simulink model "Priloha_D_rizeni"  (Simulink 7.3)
settings: Solver=ode45  StartTime=0.0  StopTime=0.7  FixedStep=0.6e-3  MaxStep=0.08e-3  RelTol=0.8e-3
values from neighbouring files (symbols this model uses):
  ILi = [0 Imax]    [Priloha_B_motor1_parametry.m]    (also in Priloha_C_motor2_parametry.m)
  Im = Psim / Ldi(1)    [Priloha_B_motor1_parametry.m]    (also in Priloha_C_motor2_parametry.m)
  Imax = 8    [Priloha_B_motor1_parametry.m]    (also in Priloha_C_motor2_parametry.m)
  J = 7e-3    (= 0.007)    [Priloha_B_motor1_parametry.m]    (also in Priloha_C_motor2_parametry.m)
  Kiid = 1 / (KM * 2 * tausigmaid / Rs)    (= 1975)    [Priloha_B_motor1_parametry.m]    (also in Priloha_C_motor2_parametry.m)
  Kiiq = 1 / (KM * 2 * tausigmaiq / Rs)    (= 1975)    [Priloha_B_motor1_parametry.m]    (also in Priloha_C_motor2_parametry.m)
  Kiwq = 1 / (Psim * p * 8 * (2 * tausigmaiq)^2 / J)    (= 306.115309264)    [Priloha_B_motor1_parametry.m]    (also in Priloha_C_motor2_parametry.m = 402.854511971)
  KM = 1    [Priloha_B_motor1_parametry.m]    (also in Priloha_C_motor2_parametry.m)
  Kpid = Ldi(1) / (KM * 2 * tausigmaid)    [Priloha_B_motor1_parametry.m]    (also in Priloha_C_motor2_parametry.m)
  Kpiq = Lqi(1) / (KM * 2 * tausigmaiq)    [Priloha_B_motor1_parametry.m]    (also in Priloha_C_motor2_parametry.m)
  Kpwq = 4 / (Psim * p * 8 * (2 * tausigmaiq) / J)    (= 2.44892247411)    [Priloha_B_motor1_parametry.m]    (also in Priloha_C_motor2_parametry.m = 3.22283609576)
  Ld = 22.5e-3    (= 0.0225)    [Priloha_B_motor1_parametry.m]    (also in Priloha_C_motor2_parametry.m)
  Ldi = [Ldi Ldi]    [Priloha_B_motor1_parametry.m]    (also in Priloha_C_motor2_parametry.m)
  Lq = 54e-3    (= 0.054)    [Priloha_B_motor1_parametry.m]    (also in Priloha_C_motor2_parametry.m)
  Lqi = [Lqi Lqi]    [Priloha_B_motor1_parametry.m]    (also in Priloha_C_motor2_parametry.m)
  p = 3    [Priloha_B_motor1_parametry.m]    (also in Priloha_C_motor2_parametry.m)
  Psim = 238.2e-3    (= 0.2382)    [Priloha_B_motor1_parametry.m]    (also in Priloha_C_motor2_parametry.m = 0.181)
  Rs = 3.95    [Priloha_B_motor1_parametry.m]    (also in Priloha_C_motor2_parametry.m)
  tausigmaid = 1 / fM    (= 0.001)    [Priloha_B_motor1_parametry.m]    (also in Priloha_C_motor2_parametry.m)
  tausigmaiq = 1 / fM    (= 0.001)    [Priloha_B_motor1_parametry.m]    (also in Priloha_C_motor2_parametry.m)
  Umax = 115    [Priloha_B_motor1_parametry.m]    (also in Priloha_C_motor2_parametry.m)
undefined symbols (not defined in the file or in its folder): Floor, magnitude
libraries: simulink x21
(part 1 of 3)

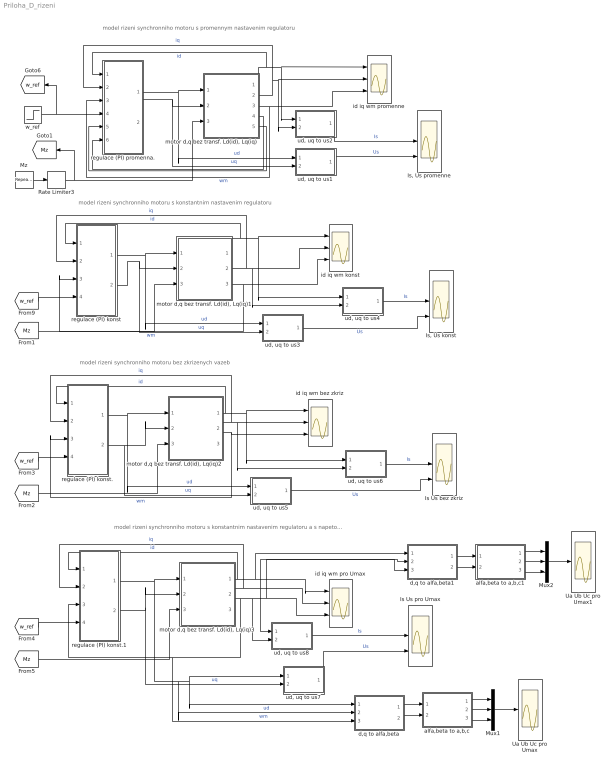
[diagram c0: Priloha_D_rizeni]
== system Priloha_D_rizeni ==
  note: model rizeni synchronniho motoru s promennym nastavenim regulatoru
  note: model rizeni synchronniho motoru s konstantnim nastavenim regulatoru
  note: model rizeni synchronniho motoru bez zkrizenych vazeb
  note: model rizeni synchronniho motoru s konstantnim nastavenim regulatoru a s napetovym omezenim
  Is Us bez zkriz : Scope  NumInputPorts=3
  Is Us pro Umax : Scope  NumInputPorts=3
  "Is, Us konst" : Scope  NumInputPorts=3
  "Is, Us promenne" : Scope  NumInputPorts=3
  Mux1 : Mux  Inputs=3
  Mux2 : Mux  Inputs=3
  Mz : simulink/Sources/Repeating Sequence Stair  SystemSampleTime=-1  OutValues=[0 0 0 4.0 4.0 4.0 0 0]  tsamp=0.1  OutMin=[]  OutMax=[]  OutDataTypeStr=double  OutputDataTypeScalingMode=Specify via dialog  OutDataType=double  ConRadixGroup=Best Precision: Vector-wise  OutScaling=2^-12
  Rate Limiter3 : RateLimiter  RisingSlewLimit=1000  FallingSlewLimit=-200000
  Ua Ub Uc pro Umax : Scope  NumInputPorts=3
  Ua Ub Uc pro Umax1 : Scope  NumInputPorts=3
  alfa,beta to a,b,c : Subsystem
  alfa,beta to a,b,c1 : Subsystem
  d,q to alfa,beta : Subsystem
  d,q to alfa,beta1 : Subsystem
  id iq wm bez zkriz : Scope  NumInputPorts=3
  id iq wm konst : Scope  NumInputPorts=3
  id iq wm pro Umax : Scope  NumInputPorts=3
  id iq wm promenne : Scope  NumInputPorts=3
  "motor d,q bez transf. Ld(id), Lq(iq)" : Subsystem
  "motor d,q bez transf. Ld(id), Lq(iq)1" : Subsystem
  "motor d,q bez transf. Ld(id), Lq(iq)2" : Subsystem
  "motor d,q bez transf. Ld(id), Lq(iq)3" : Subsystem
  regulace (PI) konst : Subsystem
  regulace (PI) konst. : Subsystem
  regulace (PI) konst.1 : Subsystem
  regulace (PI) promenna. : Subsystem
  "ud, uq to us1" : Subsystem
  "ud, uq to us2" : Subsystem
  "ud, uq to us3" : Subsystem
  "ud, uq to us4" : Subsystem
  "ud, uq to us5" : Subsystem
  "ud, uq to us6" : Subsystem
  "ud, uq to us7" : Subsystem
  "ud, uq to us8" : Subsystem
  w_ref : Step  Time=0.01  After=130  SampleTime=0
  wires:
  "ud, uq to us2"/1(is) -> "Is, Us promenne"/2  "Is"
  "motor d,q bez transf. Ld(id), Lq(iq)"/1(id) -> regulace (PI) promenna./1(id1), id iq wm promenne/1, "ud, uq to us2"/1(id)  "id"
  "motor d,q bez transf. Ld(id), Lq(iq)"/2(iq) -> regulace (PI) promenna./2(iq1), id iq wm promenne/2, "ud, uq to us2"/2(iq)  "iq"
  "motor d,q bez transf. Ld(id), Lq(iq)"/3(wm) -> id iq wm promenne/3, regulace (PI) promenna./3(wm2)  "wm"
  regulace (PI) promenna./1(ud) -> "motor d,q bez transf. Ld(id), Lq(iq)"/1(ud), "ud, uq to us1"/1(ud)  "ud"
  regulace (PI) promenna./2(uq) -> "motor d,q bez transf. Ld(id), Lq(iq)"/2(uq), "ud, uq to us1"/2(uq)  "uq"
  "ud, uq to us1"/1(us) -> "Is, Us promenne"/3  "Us"
  "motor d,q bez transf. Ld(id), Lq(iq)"/4(Ld) -> regulace (PI) promenna./6(Ld)
  "motor d,q bez transf. Ld(id), Lq(iq)"/5(Lq) -> regulace (PI) promenna./5(Lq)
  w_ref/1 -> regulace (PI) promenna./4(w_ref), [w_ref]
  Mz/1 -> Rate Limiter3/1
  Rate Limiter3/1 -> "motor d,q bez transf. Ld(id), Lq(iq)"/3(Mm), [Mz]
  "ud, uq to us4"/1(is) -> "Is, Us konst"/2  "Is"
  "motor d,q bez transf. Ld(id), Lq(iq)1"/1(id) -> regulace (PI) konst/1(id1), id iq wm konst/1, "ud, uq to us4"/1(id)  "id"
  "motor d,q bez transf. Ld(id), Lq(iq)1"/2(iq) -> id iq wm konst/2, "ud, uq to us4"/2(iq), regulace (PI) konst/2(iq1)  "iq"
  "motor d,q bez transf. Ld(id), Lq(iq)1"/3(wm) -> regulace (PI) konst/3(wm2), id iq wm konst/3  "wm"
  regulace (PI) konst/1(ud) -> "motor d,q bez transf. Ld(id), Lq(iq)1"/1(ud), "ud, uq to us3"/1(ud)  "ud"
  regulace (PI) konst/2(uq) -> "motor d,q bez transf. Ld(id), Lq(iq)1"/2(uq), "ud, uq to us3"/2(uq)  "uq"
  "ud, uq to us3"/1(us) -> "Is, Us konst"/3  "Us"
  [w_ref] -> regulace (PI) konst/4(w_ref)
  [Mz] -> "motor d,q bez transf. Ld(id), Lq(iq)1"/3(Mm)
  "ud, uq to us6"/1(is) -> Is Us bez zkriz/2  "Is"
  "motor d,q bez transf. Ld(id), Lq(iq)2"/1(id) -> id iq wm bez zkriz/1, "ud, uq to us6"/1(id), regulace (PI) konst./1(id)  "id"
  "motor d,q bez transf. Ld(id), Lq(iq)2"/2(iq) -> id iq wm bez zkriz/2, "ud, uq to us6"/2(iq), regulace (PI) konst./2(iq)  "iq"
  "motor d,q bez transf. Ld(id), Lq(iq)2"/3(wm) -> regulace (PI) konst./3(wm), id iq wm bez zkriz/3  "wm"
  regulace (PI) konst./1(ud) -> "motor d,q bez transf. Ld(id), Lq(iq)2"/1(ud), "ud, uq to us5"/1(ud)  "ud"
  regulace (PI) konst./2(uq) -> "motor d,q bez transf. Ld(id), Lq(iq)2"/2(uq), "ud, uq to us5"/2(uq)  "uq"
  "ud, uq to us5"/1(us) -> Is Us bez zkriz/3  "Us"
  [Mz] -> "motor d,q bez transf. Ld(id), Lq(iq)2"/3(Mm)
  [w_ref] -> regulace (PI) konst./4(w_ref)
  "ud, uq to us8"/1(is) -> Is Us pro Umax/2  "Is"
  "motor d,q bez transf. Ld(id), Lq(iq)3"/1(id) -> regulace (PI) konst.1/1(id1), id iq wm pro Umax/1, d,q to alfa,beta1/1(d)  "id"
  "motor d,q bez transf. Ld(id), Lq(iq)3"/2(iq) -> id iq wm pro Umax/2, "ud, uq to us8"/1(id), d,q to alfa,beta1/2(q), regulace (PI) konst.1/2(iq1)  "iq"
  "motor d,q bez transf. Ld(id), Lq(iq)3"/3(wm) -> "ud, uq to us8"/2(iq), id iq wm pro Umax/3, d,q to alfa,beta1/3(wm), regulace (PI) konst.1/3(wm2), d,q to alfa,beta/3(wm)  "wm"
  "ud, uq to us7"/1(us) -> Is Us pro Umax/3  "Us"
  d,q to alfa,beta/1(alfa) -> alfa,beta to a,b,c/1(alfa)
  d,q to alfa,beta/2(beta) -> alfa,beta to a,b,c/2(beta)
  alfa,beta to a,b,c/1(a) -> Mux1/1
  alfa,beta to a,b,c/2(b) -> Mux1/2
  alfa,beta to a,b,c/3(c) -> Mux1/3
  Mux1/1 -> Ua Ub Uc pro Umax/2
  regulace (PI) konst.1/1(ud) -> "motor d,q bez transf. Ld(id), Lq(iq)3"/1(ud), "ud, uq to us7"/1(ud), d,q to alfa,beta/1(d), d,q to alfa,beta/2(q)  "ud"
  regulace (PI) konst.1/2(uq) -> "motor d,q bez transf. Ld(id), Lq(iq)3"/2(uq), "ud, uq to us7"/2(uq)  "uq"
  [w_ref] -> regulace (PI) konst.1/4(w_ref)
  [Mz] -> "motor d,q bez transf. Ld(id), Lq(iq)3"/3(Mm)
  d,q to alfa,beta1/1(alfa) -> alfa,beta to a,b,c1/1(alfa)
  d,q to alfa,beta1/2(beta) -> alfa,beta to a,b,c1/2(beta)
  alfa,beta to a,b,c1/1(a) -> Mux2/1
  alfa,beta to a,b,c1/2(b) -> Mux2/2
  alfa,beta to a,b,c1/3(c) -> Mux2/3
  Mux2/1 -> Ua Ub Uc pro Umax1/2

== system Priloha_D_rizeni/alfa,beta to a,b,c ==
  note: transformace alfa, beta do a, b, c
  alfa : Inport  OutDataType=fixdt(1, 16)  OutScaling=2^0
  beta : Inport  Port=2  OutDataType=fixdt(1, 16)  OutScaling=2^0
  Add1 : Sum  Inputs=--  OutDataType=fixdt(1, 16)  OutScaling=2^-10
  Add5 : Sum  Inputs=-+  OutDataType=fixdt(1, 16)  OutScaling=2^-10
  Gain1 : Gain  Gain=1/2  ParameterDataType=fixdt(1, 16)  ParameterScaling=2^0  OutDataType=fixdt(1, 16)  OutScaling=2^0
  Gain2 : Gain  Gain=sqrt(3)/2  ParameterDataType=fixdt(1, 16)  ParameterScaling=2^0  OutDataType=fixdt(1, 16)  OutScaling=2^0
  a : Outport  OutDataType=fixdt(1, 16)  OutScaling=2^0
  b : Outport  Port=2  OutDataType=fixdt(1, 16)  OutScaling=2^0
  c : Outport  Port=3  OutDataType=fixdt(1, 16)  OutScaling=2^0
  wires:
  alfa/1 -> a/1, Gain1/1
  Gain1/1 -> Add5/1, Add1/1
  Add5/1 -> b/1
  beta/1 -> Gain2/1
  Add1/1 -> c/1
  Gain2/1 -> Add5/2, Add1/2

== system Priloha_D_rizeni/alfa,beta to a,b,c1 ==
  note: transformace alfa, beta do a, b, c
  alfa : Inport  OutDataType=fixdt(1, 16)  OutScaling=2^0
  beta : Inport  Port=2  OutDataType=fixdt(1, 16)  OutScaling=2^0
  Add1 : Sum  Inputs=--  OutDataType=fixdt(1, 16)  OutScaling=2^-10
  Add5 : Sum  Inputs=-+  OutDataType=fixdt(1, 16)  OutScaling=2^-10
  Gain1 : Gain  Gain=1/2  ParameterDataType=fixdt(1, 16)  ParameterScaling=2^0  OutDataType=fixdt(1, 16)  OutScaling=2^0
  Gain2 : Gain  Gain=sqrt(3)/2  ParameterDataType=fixdt(1, 16)  ParameterScaling=2^0  OutDataType=fixdt(1, 16)  OutScaling=2^0
  a : Outport  OutDataType=fixdt(1, 16)  OutScaling=2^0
  b : Outport  Port=2  OutDataType=fixdt(1, 16)  OutScaling=2^0
  c : Outport  Port=3  OutDataType=fixdt(1, 16)  OutScaling=2^0
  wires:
  alfa/1 -> a/1, Gain1/1
  Gain1/1 -> Add5/1, Add1/1
  Add5/1 -> b/1
  beta/1 -> Gain2/1
  Add1/1 -> c/1
  Gain2/1 -> Add5/2, Add1/2

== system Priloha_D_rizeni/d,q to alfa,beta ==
  note: transformace d,q do alfa, beta
  d : Inport  OutDataType=fixdt(1, 16)  OutScaling=2^0
  q : Inport  Port=2  OutDataType=fixdt(1, 16)  OutScaling=2^0
  wm : Inport  Port=3  OutDataType=fixdt(1, 16)  OutScaling=2^0
  Add1 : Sum  OutDataType=fixdt(1, 16)  OutScaling=2^-10
  Add5 : Sum  Inputs=+-  OutDataType=fixdt(1, 16)  OutScaling=2^-10
  Gain5 : Gain  Gain=p  ParameterDataType=fixdt(1, 16)  ParameterScaling=2^0  OutDataType=fixdt(1, 16)  OutScaling=2^0
  Integrator4 : Integrator
  Product{1..4} (4 alike) : Product  OutDataType=fixdt(1, 16)  OutScaling=2^0
  cos : Trigonometry  Operator=cos
  sin : Trigonometry
  alfa : Outport  OutDataType=fixdt(1, 16)  OutScaling=2^0
  beta : Outport  Port=2  OutDataType=fixdt(1, 16)  OutScaling=2^0
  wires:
  Add5/1 -> alfa/1
  Product1/1 -> Add5/1
  d/1 -> Product4/2, Product1/1
  q/1 -> Product3/2, Product2/1
  Product2/1 -> Add5/2
  Add1/1 -> beta/1
  wm/1 -> Gain5/1  "wm"
  Gain5/1 -> Integrator4/1  "we"
  Integrator4/1 -> sin/1, cos/1
  sin/1 -> Product4/1, Product2/2
  cos/1 -> Product1/2, Product3/1
  Product4/1 -> Add1/1
  Product3/1 -> Add1/2

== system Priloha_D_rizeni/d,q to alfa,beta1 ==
  note: transformace d,q do alfa, beta
  d : Inport  OutDataType=fixdt(1, 16)  OutScaling=2^0
  q : Inport  Port=2  OutDataType=fixdt(1, 16)  OutScaling=2^0
  wm : Inport  Port=3  OutDataType=fixdt(1, 16)  OutScaling=2^0
  Add1 : Sum  OutDataType=fixdt(1, 16)  OutScaling=2^-10
  Add5 : Sum  Inputs=+-  OutDataType=fixdt(1, 16)  OutScaling=2^-10
  Gain5 : Gain  Gain=p  ParameterDataType=fixdt(1, 16)  ParameterScaling=2^0  OutDataType=fixdt(1, 16)  OutScaling=2^0
  Integrator4 : Integrator
  Product{1..4} (4 alike) : Product  OutDataType=fixdt(1, 16)  OutScaling=2^0
  cos : Trigonometry  Operator=cos
  sin : Trigonometry
  alfa : Outport  OutDataType=fixdt(1, 16)  OutScaling=2^0
  beta : Outport  Port=2  OutDataType=fixdt(1, 16)  OutScaling=2^0
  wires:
  Add5/1 -> alfa/1
  Product1/1 -> Add5/1
  d/1 -> Product4/2, Product1/1
  q/1 -> Product3/2, Product2/1
  Product2/1 -> Add5/2
  Add1/1 -> beta/1
  wm/1 -> Gain5/1  "wm"
  Gain5/1 -> Integrator4/1  "we"
  Integrator4/1 -> sin/1, cos/1
  sin/1 -> Product4/1, Product2/2
  cos/1 -> Product1/2, Product3/1
  Product4/1 -> Add1/1
  Product3/1 -> Add1/2

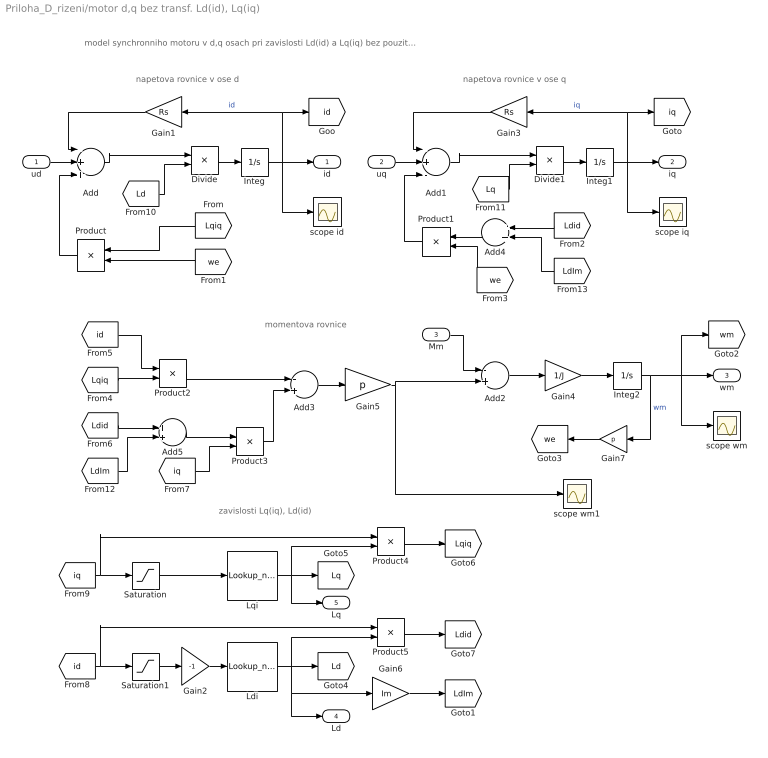
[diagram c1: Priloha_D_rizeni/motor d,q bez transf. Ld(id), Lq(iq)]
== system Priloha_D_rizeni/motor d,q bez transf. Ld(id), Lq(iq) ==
  note: zavislosti Lq(iq), Ld(id)
  note: momentova rovnice
  note: napetova rovnice v ose q
  note: napetova rovnice v ose d
  note: model synchronniho motoru v d,q osach pri zavislosti Ld(id) a Lq(iq) bez pouziti transformace (v momentove rovnici neni koeficient 3/2)
  ud : Inport  OutDataType=fixdt(1, 16)  OutScaling=2^0
  uq : Inport  Port=2  OutDataType=fixdt(1, 16)  OutScaling=2^0
  Mm : Inport  Port=3  OutDataType=fixdt(1, 16)  OutScaling=2^0
  Add : Sum  Inputs=-++  OutDataType=fixdt(1, 16)  OutScaling=2^-10
  Add1 : Sum  Inputs=-+-  OutDataType=fixdt(1, 16)  OutScaling=2^-10
  Add2 : Sum  Inputs=-+  OutDataType=fixdt(1, 16)  OutScaling=2^-10
  Add3 : Sum  Inputs=-+  OutDataType=fixdt(1, 16)  OutScaling=2^-10
  Add4 : Sum  OutDataType=fixdt(1, 16)  OutScaling=2^-10
  Add5 : Sum  OutDataType=fixdt(1, 16)  OutScaling=2^-10
  Divide : Product  Inputs=*/  OutDataType=fixdt(1, 16)  OutScaling=2^-10
  Divide1 : Product  Inputs=*/  OutDataType=fixdt(1, 16)  OutScaling=2^-10
  Gain1 : Gain  Gain=Rs  ParameterDataType=fixdt(1, 16)  ParameterScaling=2^0  OutDataType=fixdt(1, 16)  OutScaling=2^0
  Gain2 : Gain  Gain=-1  ParameterDataType=fixdt(1, 16)  ParameterScaling=2^0  OutDataType=fixdt(1, 16)  OutScaling=2^0
  Gain3 : Gain  Gain=Rs  ParameterDataType=fixdt(1, 16)  ParameterScaling=2^0  OutDataType=fixdt(1, 16)  OutScaling=2^0
  Gain4 : Gain  Gain=1/J  ParameterDataType=fixdt(1, 16)  ParameterScaling=2^0  OutDataType=fixdt(1, 16)  OutScaling=2^0
  Gain5 : Gain  Gain=p  ParameterDataType=fixdt(1, 16)  ParameterScaling=2^0  OutDataType=fixdt(1, 16)  OutScaling=2^0
  Gain6 : Gain  Gain=Im  ParameterDataType=fixdt(1, 16)  ParameterScaling=2^0  OutDataType=fixdt(1, 16)  OutScaling=2^0
  Gain7 : Gain  Gain=p  ParameterDataType=fixdt(1, 16)  ParameterScaling=2^0  OutDataType=fixdt(1, 16)  OutScaling=2^0
  Integ : Integrator
  Integ1 : Integrator
  Integ2 : Integrator
  Ldi : Lookup_n-D  NumberOfTableDimensions=1  BreakpointsForDimension1=[ILi]  Table=[Ldi]
  Lqi : Lookup_n-D  NumberOfTableDimensions=1  BreakpointsForDimension1=[ILi]  Table=[Lqi]
  Product{,1..5} (6 alike) : Product  OutDataType=fixdt(1, 16)  OutScaling=2^0
  Saturation : Saturate  UpperLimit=Imax  LowerLimit=ILi(1)  OutDataType=fixdt(1, 16)  OutScaling=2^0
  Saturation1 : Saturate  UpperLimit=ILi(1)  LowerLimit=-Imax  OutDataType=fixdt(1, 16)  OutScaling=2^0
  scope id : Scope
  scope iq : Scope
  scope wm : Scope
  scope wm1 : Scope
  id : Outport  OutDataType=fixdt(1, 16)  OutScaling=2^0
  iq : Outport  Port=2  OutDataType=fixdt(1, 16)  OutScaling=2^0
  wm : Outport  Port=3  OutDataType=fixdt(1, 16)  OutScaling=2^0
  Ld : Outport  Port=4  OutDataType=fixdt(1, 16)  OutScaling=2^0
  Lq : Outport  Port=5  OutDataType=fixdt(1, 16)  OutScaling=2^0
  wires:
  [LdIm] -> Add4/2
  [LdIm] -> Add5/2
  Gain6/1 -> [LdIm]
  Gain2/1 -> Ldi/1
  [Lq] -> Divide1/2
  Add1/1 -> Divide1/1
  [Lqiq] -> Product/1
  Divide1/1 -> Integ1/1
  [Ld] -> Divide/2
  Add/1 -> Divide/1
  Divide/1 -> Integ/1
  Product5/1 -> [Ldid]
  Product4/1 -> [Lqiq]
  Ldi/1 -> Product5/2, [Ld], Gain6/1, Ld/1
  [id] -> Product5/1, Saturation1/1
  Lqi/1 -> Product4/2, [Lq], Lq/1
  [iq] -> Product4/1, Saturation/1
  Saturation1/1 -> Gain2/1
  Saturation/1 -> Lqi/1
  [we] -> Product/2
  Product/1 -> Add/3
  [we] -> Product1/2
  Product1/1 -> Add1/3
  Product3/1 -> Add3/2
  [iq] -> Product3/2
  Add5/1 -> Product3/1
  [Ldid] -> Add5/1
  Product2/1 -> Add3/1
  [id] -> Product2/1
  [Lqiq] -> Product2/2
  Add4/1 -> Product1/1
  [Ldid] -> Add4/1
  Gain7/1 -> [we]
  Add3/1 -> Gain5/1
  Mm/1 -> Add2/1
  Gain5/1 -> scope wm1/1, Add2/2
  Add2/1 -> Gain4/1
  Gain4/1 -> Integ2/1
  Integ2/1 -> Gain7/1, [wm], scope wm/1, wm/1  "wm"
  uq/1 -> Add1/2
  Gain3/1 -> Add1/1
  Integ1/1 -> Gain3/1, [iq], iq/1, scope iq/1  "iq"
  ud/1 -> Add/2
  Gain1/1 -> Add/1
  Integ/1 -> Gain1/1, [id], scope id/1, id/1  "id"

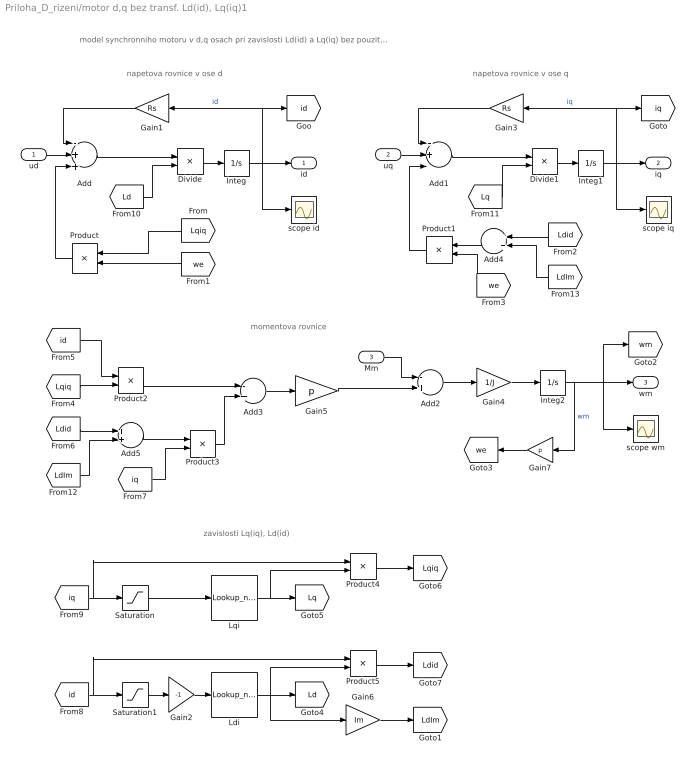
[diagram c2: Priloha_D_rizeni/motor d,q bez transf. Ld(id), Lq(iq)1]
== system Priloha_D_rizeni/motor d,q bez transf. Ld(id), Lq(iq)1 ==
  note: zavislosti Lq(iq), Ld(id)
  note: momentova rovnice
  note: napetova rovnice v ose q
  note: napetova rovnice v ose d
  note: model synchronniho motoru v d,q osach pri zavislosti Ld(id) a Lq(iq) bez pouziti transformace (v momentove rovnici neni koeficient 3/2)
  ud : Inport  OutDataType=fixdt(1, 16)  OutScaling=2^0
  uq : Inport  Port=2  OutDataType=fixdt(1, 16)  OutScaling=2^0
  Mm : Inport  Port=3  OutDataType=fixdt(1, 16)  OutScaling=2^0
  Add : Sum  Inputs=-++  OutDataType=fixdt(1, 16)  OutScaling=2^-10
  Add1 : Sum  Inputs=-+-  OutDataType=fixdt(1, 16)  OutScaling=2^-10
  Add2 : Sum  Inputs=-+  OutDataType=fixdt(1, 16)  OutScaling=2^-10
  Add3 : Sum  Inputs=-+  OutDataType=fixdt(1, 16)  OutScaling=2^-10
  Add4 : Sum  OutDataType=fixdt(1, 16)  OutScaling=2^-10
  Add5 : Sum  OutDataType=fixdt(1, 16)  OutScaling=2^-10
  Divide : Product  Inputs=*/  OutDataType=fixdt(1, 16)  OutScaling=2^-10
  Divide1 : Product  Inputs=*/  OutDataType=fixdt(1, 16)  OutScaling=2^-10
  Gain1 : Gain  Gain=Rs  ParameterDataType=fixdt(1, 16)  ParameterScaling=2^0  OutDataType=fixdt(1, 16)  OutScaling=2^0
  Gain2 : Gain  Gain=-1  ParameterDataType=fixdt(1, 16)  ParameterScaling=2^0  OutDataType=fixdt(1, 16)  OutScaling=2^0
  Gain3 : Gain  Gain=Rs  ParameterDataType=fixdt(1, 16)  ParameterScaling=2^0  OutDataType=fixdt(1, 16)  OutScaling=2^0
  Gain4 : Gain  Gain=1/J  ParameterDataType=fixdt(1, 16)  ParameterScaling=2^0  OutDataType=fixdt(1, 16)  OutScaling=2^0
  Gain5 : Gain  Gain=p  ParameterDataType=fixdt(1, 16)  ParameterScaling=2^0  OutDataType=fixdt(1, 16)  OutScaling=2^0
  Gain6 : Gain  Gain=Im  ParameterDataType=fixdt(1, 16)  ParameterScaling=2^0  OutDataType=fixdt(1, 16)  OutScaling=2^0
  Gain7 : Gain  Gain=p  ParameterDataType=fixdt(1, 16)  ParameterScaling=2^0  OutDataType=fixdt(1, 16)  OutScaling=2^0
  Integ : Integrator
  Integ1 : Integrator
  Integ2 : Integrator
  Ldi : Lookup_n-D  NumberOfTableDimensions=1  BreakpointsForDimension1=[ILi]  Table=[Ldi]
  Lqi : Lookup_n-D  NumberOfTableDimensions=1  BreakpointsForDimension1=[ILi]  Table=[Lqi]
  Product{,1..5} (6 alike) : Product  OutDataType=fixdt(1, 16)  OutScaling=2^0
  Saturation : Saturate  UpperLimit=Imax  LowerLimit=ILi(1)  OutDataType=fixdt(1, 16)  OutScaling=2^0
  Saturation1 : Saturate  UpperLimit=ILi(1)  LowerLimit=-Imax  OutDataType=fixdt(1, 16)  OutScaling=2^0
  scope id : Scope
  scope iq : Scope
  scope wm : Scope
  id : Outport  OutDataType=fixdt(1, 16)  OutScaling=2^0
  iq : Outport  Port=2  OutDataType=fixdt(1, 16)  OutScaling=2^0
  wm : Outport  Port=3  OutDataType=fixdt(1, 16)  OutScaling=2^0
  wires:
  [LdIm] -> Add4/2
  [LdIm] -> Add5/2
  Gain6/1 -> [LdIm]
  Gain2/1 -> Ldi/1
  [Lq] -> Divide1/2
  Add1/1 -> Divide1/1
  [Lqiq] -> Product/1
  Divide1/1 -> Integ1/1
  [Ld] -> Divide/2
  Add/1 -> Divide/1
  Divide/1 -> Integ/1
  Product5/1 -> [Ldid]
  Product4/1 -> [Lqiq]
  Ldi/1 -> Gain6/1, Product5/2, [Ld]
  [id] -> Product5/1, Saturation1/1
  Lqi/1 -> Product4/2, [Lq]
  [iq] -> Product4/1, Saturation/1
  Saturation1/1 -> Gain2/1
  Saturation/1 -> Lqi/1
  [we] -> Product/2
  Product/1 -> Add/3
  [we] -> Product1/2
  Product1/1 -> Add1/3
  Product3/1 -> Add3/2
  [iq] -> Product3/2
  Add5/1 -> Product3/1
  [Ldid] -> Add5/1
  Product2/1 -> Add3/1
  [id] -> Product2/1
  [Lqiq] -> Product2/2
  Add4/1 -> Product1/1
  [Ldid] -> Add4/1
  Gain7/1 -> [we]
  Add3/1 -> Gain5/1
  Mm/1 -> Add2/1
  Gain5/1 -> Add2/2
  Add2/1 -> Gain4/1
  Gain4/1 -> Integ2/1
  Integ2/1 -> Gain7/1, [wm], scope wm/1, wm/1  "wm"
  uq/1 -> Add1/2
  Gain3/1 -> Add1/1
  Integ1/1 -> Gain3/1, [iq], iq/1, scope iq/1  "iq"
  ud/1 -> Add/2
  Gain1/1 -> Add/1
  Integ/1 -> Gain1/1, [id], scope id/1, id/1  "id"

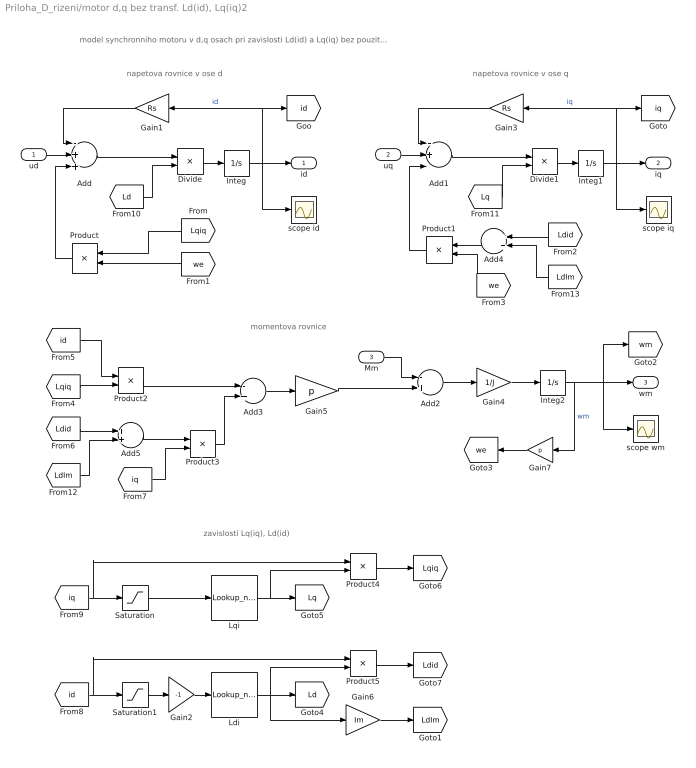
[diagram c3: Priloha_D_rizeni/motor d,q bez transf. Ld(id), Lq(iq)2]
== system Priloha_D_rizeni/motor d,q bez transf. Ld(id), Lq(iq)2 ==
  note: zavislosti Lq(iq), Ld(id)
  note: momentova rovnice
  note: napetova rovnice v ose q
  note: napetova rovnice v ose d
  note: model synchronniho motoru v d,q osach pri zavislosti Ld(id) a Lq(iq) bez pouziti transformace (v momentove rovnici neni koeficient 3/2)
  ud : Inport  OutDataType=fixdt(1, 16)  OutScaling=2^0
  uq : Inport  Port=2  OutDataType=fixdt(1, 16)  OutScaling=2^0
  Mm : Inport  Port=3  OutDataType=fixdt(1, 16)  OutScaling=2^0
  Add : Sum  Inputs=-++  OutDataType=fixdt(1, 16)  OutScaling=2^-10
  Add1 : Sum  Inputs=-+-  OutDataType=fixdt(1, 16)  OutScaling=2^-10
  Add2 : Sum  Inputs=-+  OutDataType=fixdt(1, 16)  OutScaling=2^-10
  Add3 : Sum  Inputs=-+  OutDataType=fixdt(1, 16)  OutScaling=2^-10
  Add4 : Sum  OutDataType=fixdt(1, 16)  OutScaling=2^-10
  Add5 : Sum  OutDataType=fixdt(1, 16)  OutScaling=2^-10
  Divide : Product  Inputs=*/  OutDataType=fixdt(1, 16)  OutScaling=2^-10
  Divide1 : Product  Inputs=*/  OutDataType=fixdt(1, 16)  OutScaling=2^-10
  Gain1 : Gain  Gain=Rs  ParameterDataType=fixdt(1, 16)  ParameterScaling=2^0  OutDataType=fixdt(1, 16)  OutScaling=2^0
  Gain2 : Gain  Gain=-1  ParameterDataType=fixdt(1, 16)  ParameterScaling=2^0  OutDataType=fixdt(1, 16)  OutScaling=2^0
  Gain3 : Gain  Gain=Rs  ParameterDataType=fixdt(1, 16)  ParameterScaling=2^0  OutDataType=fixdt(1, 16)  OutScaling=2^0
  Gain4 : Gain  Gain=1/J  ParameterDataType=fixdt(1, 16)  ParameterScaling=2^0  OutDataType=fixdt(1, 16)  OutScaling=2^0
  Gain5 : Gain  Gain=p  ParameterDataType=fixdt(1, 16)  ParameterScaling=2^0  OutDataType=fixdt(1, 16)  OutScaling=2^0
  Gain6 : Gain  Gain=Im  ParameterDataType=fixdt(1, 16)  ParameterScaling=2^0  OutDataType=fixdt(1, 16)  OutScaling=2^0
  Gain7 : Gain  Gain=p  ParameterDataType=fixdt(1, 16)  ParameterScaling=2^0  OutDataType=fixdt(1, 16)  OutScaling=2^0
  Integ : Integrator
  Integ1 : Integrator
  Integ2 : Integrator
  Ldi : Lookup_n-D  NumberOfTableDimensions=1  BreakpointsForDimension1=[ILi]  Table=[Ldi]
  Lqi : Lookup_n-D  NumberOfTableDimensions=1  BreakpointsForDimension1=[ILi]  Table=[Lqi]
  Product{,1..5} (6 alike) : Product  OutDataType=fixdt(1, 16)  OutScaling=2^0
  Saturation : Saturate  UpperLimit=Imax  LowerLimit=ILi(1)  OutDataType=fixdt(1, 16)  OutScaling=2^0
  Saturation1 : Saturate  UpperLimit=ILi(1)  LowerLimit=-Imax  OutDataType=fixdt(1, 16)  OutScaling=2^0
  scope id : Scope
  scope iq : Scope
  scope wm : Scope
  id : Outport  OutDataType=fixdt(1, 16)  OutScaling=2^0
  iq : Outport  Port=2  OutDataType=fixdt(1, 16)  OutScaling=2^0
  wm : Outport  Port=3  OutDataType=fixdt(1, 16)  OutScaling=2^0
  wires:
  [LdIm] -> Add4/2
  [LdIm] -> Add5/2
  Gain6/1 -> [LdIm]
  Gain2/1 -> Ldi/1
  [Lq] -> Divide1/2
  Add1/1 -> Divide1/1
  [Lqiq] -> Product/1
  Divide1/1 -> Integ1/1
  [Ld] -> Divide/2
  Add/1 -> Divide/1
  Divide/1 -> Integ/1
  Product5/1 -> [Ldid]
  Product4/1 -> [Lqiq]
  Ldi/1 -> Gain6/1, Product5/2, [Ld]
  [id] -> Product5/1, Saturation1/1
  Lqi/1 -> Product4/2, [Lq]
  [iq] -> Product4/1, Saturation/1
  Saturation1/1 -> Gain2/1
  Saturation/1 -> Lqi/1
  [we] -> Product/2
  Product/1 -> Add/3
  [we] -> Product1/2
  Product1/1 -> Add1/3
  Product3/1 -> Add3/2
  [iq] -> Product3/2
  Add5/1 -> Product3/1
  [Ldid] -> Add5/1
  Product2/1 -> Add3/1
  [id] -> Product2/1
  [Lqiq] -> Product2/2
  Add4/1 -> Product1/1
  [Ldid] -> Add4/1
  Gain7/1 -> [we]
  Add3/1 -> Gain5/1
  Mm/1 -> Add2/1
  Gain5/1 -> Add2/2
  Add2/1 -> Gain4/1
  Gain4/1 -> Integ2/1
  Integ2/1 -> Gain7/1, [wm], scope wm/1, wm/1  "wm"
  uq/1 -> Add1/2
  Gain3/1 -> Add1/1
  Integ1/1 -> Gain3/1, [iq], iq/1, scope iq/1  "iq"
  ud/1 -> Add/2
  Gain1/1 -> Add/1
  Integ/1 -> Gain1/1, [id], scope id/1, id/1  "id"

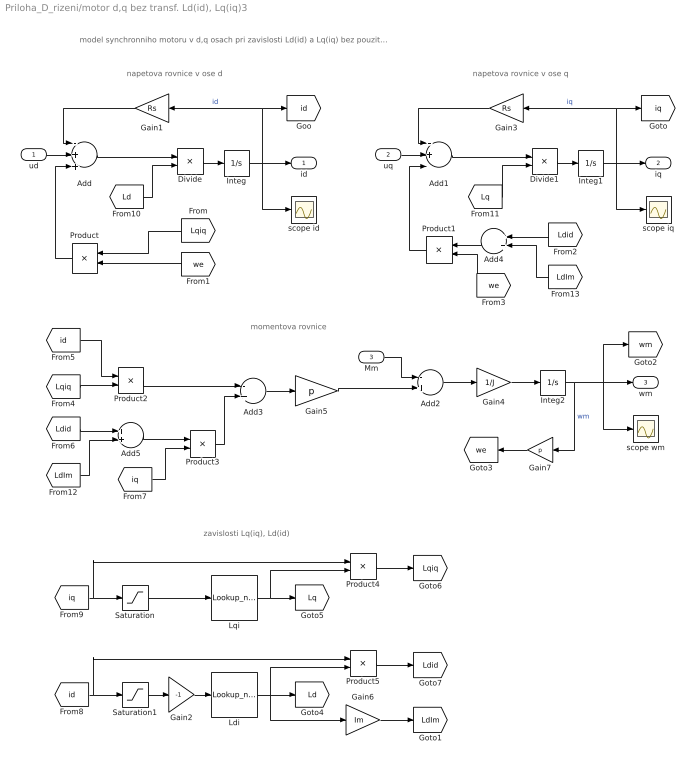
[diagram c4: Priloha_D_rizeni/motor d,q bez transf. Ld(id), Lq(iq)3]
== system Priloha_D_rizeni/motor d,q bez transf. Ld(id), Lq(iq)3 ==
  note: zavislosti Lq(iq), Ld(id)
  note: momentova rovnice
  note: napetova rovnice v ose q
  note: napetova rovnice v ose d
  note: model synchronniho motoru v d,q osach pri zavislosti Ld(id) a Lq(iq) bez pouziti transformace (v momentove rovnici neni koeficient 3/2)
  ud : Inport  OutDataType=fixdt(1, 16)  OutScaling=2^0
  uq : Inport  Port=2  OutDataType=fixdt(1, 16)  OutScaling=2^0
  Mm : Inport  Port=3  OutDataType=fixdt(1, 16)  OutScaling=2^0
  Add : Sum  Inputs=-++  OutDataType=fixdt(1, 16)  OutScaling=2^-10
  Add1 : Sum  Inputs=-+-  OutDataType=fixdt(1, 16)  OutScaling=2^-10
  Add2 : Sum  Inputs=-+  OutDataType=fixdt(1, 16)  OutScaling=2^-10
  Add3 : Sum  Inputs=-+  OutDataType=fixdt(1, 16)  OutScaling=2^-10
  Add4 : Sum  OutDataType=fixdt(1, 16)  OutScaling=2^-10
  Add5 : Sum  OutDataType=fixdt(1, 16)  OutScaling=2^-10
  Divide : Product  Inputs=*/  OutDataType=fixdt(1, 16)  OutScaling=2^-10
  Divide1 : Product  Inputs=*/  OutDataType=fixdt(1, 16)  OutScaling=2^-10
  Gain1 : Gain  Gain=Rs  ParameterDataType=fixdt(1, 16)  ParameterScaling=2^0  OutDataType=fixdt(1, 16)  OutScaling=2^0
  Gain2 : Gain  Gain=-1  ParameterDataType=fixdt(1, 16)  ParameterScaling=2^0  OutDataType=fixdt(1, 16)  OutScaling=2^0
  Gain3 : Gain  Gain=Rs  ParameterDataType=fixdt(1, 16)  ParameterScaling=2^0  OutDataType=fixdt(1, 16)  OutScaling=2^0
  Gain4 : Gain  Gain=1/J  ParameterDataType=fixdt(1, 16)  ParameterScaling=2^0  OutDataType=fixdt(1, 16)  OutScaling=2^0
  Gain5 : Gain  Gain=p  ParameterDataType=fixdt(1, 16)  ParameterScaling=2^0  OutDataType=fixdt(1, 16)  OutScaling=2^0
  Gain6 : Gain  Gain=Im  ParameterDataType=fixdt(1, 16)  ParameterScaling=2^0  OutDataType=fixdt(1, 16)  OutScaling=2^0
  Gain7 : Gain  Gain=p  ParameterDataType=fixdt(1, 16)  ParameterScaling=2^0  OutDataType=fixdt(1, 16)  OutScaling=2^0
  Integ : Integrator
  Integ1 : Integrator
  Integ2 : Integrator
  Ldi : Lookup_n-D  NumberOfTableDimensions=1  BreakpointsForDimension1=[ILi]  Table=[Ldi]
  Lqi : Lookup_n-D  NumberOfTableDimensions=1  BreakpointsForDimension1=[ILi]  Table=[Lqi]
  Product{,1..5} (6 alike) : Product  OutDataType=fixdt(1, 16)  OutScaling=2^0
  Saturation : Saturate  UpperLimit=Imax  LowerLimit=ILi(1)  OutDataType=fixdt(1, 16)  OutScaling=2^0
  Saturation1 : Saturate  UpperLimit=ILi(1)  LowerLimit=-Imax  OutDataType=fixdt(1, 16)  OutScaling=2^0
  scope id : Scope
  scope iq : Scope
  scope wm : Scope
  id : Outport  OutDataType=fixdt(1, 16)  OutScaling=2^0
  iq : Outport  Port=2  OutDataType=fixdt(1, 16)  OutScaling=2^0
  wm : Outport  Port=3  OutDataType=fixdt(1, 16)  OutScaling=2^0
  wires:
  [LdIm] -> Add4/2
  [LdIm] -> Add5/2
  Gain6/1 -> [LdIm]
  Gain2/1 -> Ldi/1
  [Lq] -> Divide1/2
  Add1/1 -> Divide1/1
  [Lqiq] -> Product/1
  Divide1/1 -> Integ1/1
  [Ld] -> Divide/2
  Add/1 -> Divide/1
  Divide/1 -> Integ/1
  Product5/1 -> [Ldid]
  Product4/1 -> [Lqiq]
  Ldi/1 -> Gain6/1, Product5/2, [Ld]
  [id] -> Product5/1, Saturation1/1
  Lqi/1 -> Product4/2, [Lq]
  [iq] -> Product4/1, Saturation/1
  Saturation1/1 -> Gain2/1
  Saturation/1 -> Lqi/1
  [we] -> Product/2
  Product/1 -> Add/3
  [we] -> Product1/2
  Product1/1 -> Add1/3
  Product3/1 -> Add3/2
  [iq] -> Product3/2
  Add5/1 -> Product3/1
  [Ldid] -> Add5/1
  Product2/1 -> Add3/1
  [id] -> Product2/1
  [Lqiq] -> Product2/2
  Add4/1 -> Product1/1
  [Ldid] -> Add4/1
  Gain7/1 -> [we]
  Add3/1 -> Gain5/1
  Mm/1 -> Add2/1
  Gain5/1 -> Add2/2
  Add2/1 -> Gain4/1
  Gain4/1 -> Integ2/1
  Integ2/1 -> Gain7/1, [wm], scope wm/1, wm/1  "wm"
  uq/1 -> Add1/2
  Gain3/1 -> Add1/1
  Integ1/1 -> Gain3/1, [iq], iq/1, scope iq/1  "iq"
  ud/1 -> Add/2
  Gain1/1 -> Add/1
  Integ/1 -> Gain1/1, [id], scope id/1, id/1  "id"

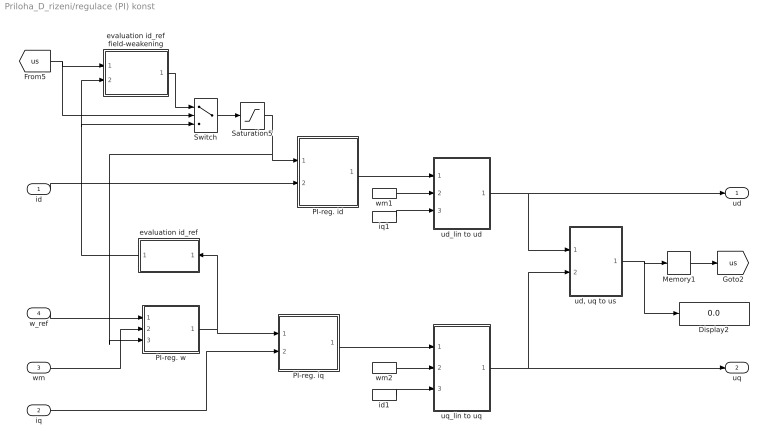
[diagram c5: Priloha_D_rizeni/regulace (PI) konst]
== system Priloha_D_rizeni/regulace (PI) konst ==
  id : Inport
  iq : Inport  Port=2
  wm : Inport  Port=3
  w_ref : Inport  Port=4
  Display2 : Display
  Memory1 : Memory  InheritSampleTime=on
  PI-reg. id : Subsystem
  PI-reg. iq : Subsystem
  PI-reg. w : Subsystem
  Saturation5 : Saturate  UpperLimit=Imax  LowerLimit=-Imax  OutDataType=fixdt(1, 16)  OutScaling=2^0
  Switch : Switch  Threshold=Umax * 0.95  OutDataType=fixdt(1, 16)  OutScaling=2^0  ZeroCross=off
  evaluation id_ref : Subsystem
  evaluation id_ref field-weakening : Subsystem
  id1 : InportShadow  Port=1  LatchByCopyingInsideSignal=off
  iq1 : InportShadow  Port=2  LatchByCopyingInsideSignal=off
  "ud, uq to us" : Subsystem
  ud_lin to ud : Subsystem
  uq_lin to uq : Subsystem
  wm1 : InportShadow  Port=3  LatchByCopyingInsideSignal=off
  wm2 : InportShadow  Port=3  LatchByCopyingInsideSignal=off
  ud : Outport  OutDataType=fixdt(1, 16)  OutScaling=2^0
  uq : Outport  Port=2  OutDataType=fixdt(1, 16)  OutScaling=2^0
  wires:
  PI-reg. w/1(iq_ref) -> PI-reg. iq/1(iq_ref), evaluation id_ref/1(iq_ref)
  w_ref/1 -> PI-reg. w/1(w_ref)
  wm/1 -> PI-reg. w/2(wm)
  evaluation id_ref/1(id_ref) -> evaluation id_ref field-weakening/2(id_mtpa), Switch/3
  "ud, uq to us"/1(us) -> Display2/1, Memory1/1
  [us] -> evaluation id_ref field-weakening/1(us), Switch/2
  id/1 -> PI-reg. id/2(id)
  iq1/1 -> ud_lin to ud/3(iq)
  iq/1 -> PI-reg. iq/2(iq)
  wm1/1 -> ud_lin to ud/2(wm)
  id1/1 -> uq_lin to uq/3(id)
  wm2/1 -> uq_lin to uq/2(wm)
  Memory1/1 -> [us]
  PI-reg. iq/1(uq1) -> uq_lin to uq/1(uq1)
  PI-reg. id/1(ud1) -> ud_lin to ud/1(ud1)
  evaluation id_ref field-weakening/1(id_ref) -> Switch/1
  Switch/1 -> Saturation5/1
  uq_lin to uq/1(uq2) -> uq/1, "ud, uq to us"/2(uq2)
  ud_lin to ud/1(ud2) -> "ud, uq to us"/1(ud2), ud/1
  Saturation5/1 -> PI-reg. id/1(id_ref), PI-reg. w/3(id_ref)

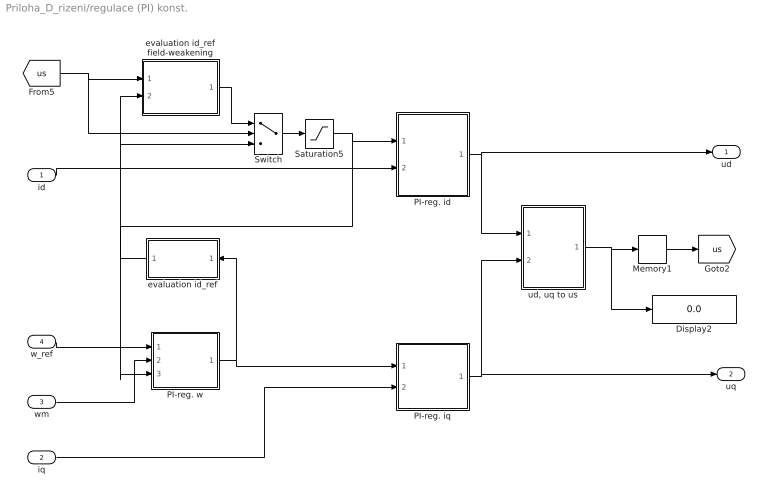
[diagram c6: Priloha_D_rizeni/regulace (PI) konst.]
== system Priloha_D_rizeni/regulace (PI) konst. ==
  id : Inport
  iq : Inport  Port=2
  wm : Inport  Port=3
  w_ref : Inport  Port=4
  Display2 : Display
  Memory1 : Memory  InheritSampleTime=on
  PI-reg. id : Subsystem
  PI-reg. iq : Subsystem
  PI-reg. w : Subsystem
  Saturation5 : Saturate  UpperLimit=Imax  LowerLimit=-Imax  OutDataType=fixdt(1, 16)  OutScaling=2^0
  Switch : Switch  Threshold=Umax * 0.95  OutDataType=fixdt(1, 16)  OutScaling=2^0  ZeroCross=off
  evaluation id_ref : Subsystem
  evaluation id_ref field-weakening : Subsystem
  "ud, uq to us" : Subsystem
  ud : Outport  OutDataType=fixdt(1, 16)  OutScaling=2^0
  uq : Outport  Port=2  OutDataType=fixdt(1, 16)  OutScaling=2^0
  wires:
  PI-reg. w/1(iq_ref) -> PI-reg. iq/1(iq_ref), evaluation id_ref/1(iq_ref)
  w_ref/1 -> PI-reg. w/1(w_ref)
  wm/1 -> PI-reg. w/2(wm)
  evaluation id_ref/1(id_ref) -> evaluation id_ref field-weakening/2(id_mtpa), Switch/3
  "ud, uq to us"/1(us) -> Display2/1, Memory1/1
  [us] -> evaluation id_ref field-weakening/1(us), Switch/2
  id/1 -> PI-reg. id/2(id)
  iq/1 -> PI-reg. iq/2(iq)
  Memory1/1 -> [us]
  evaluation id_ref field-weakening/1(id_ref) -> Switch/1
  Switch/1 -> Saturation5/1
  PI-reg. id/1(ud1) -> ud/1, "ud, uq to us"/1(ud1)
  PI-reg. iq/1(uq1) -> uq/1, "ud, uq to us"/2(uq1)
  Saturation5/1 -> PI-reg. id/1(id_ref), PI-reg. w/3(id_ref)

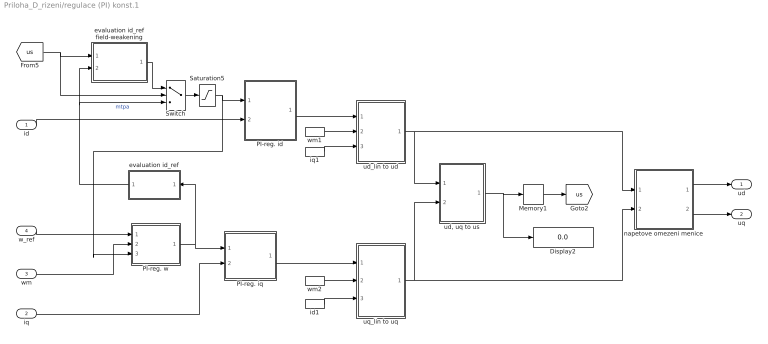
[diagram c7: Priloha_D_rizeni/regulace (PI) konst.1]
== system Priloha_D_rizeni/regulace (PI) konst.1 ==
  id : Inport
  iq : Inport  Port=2
  wm : Inport  Port=3
  w_ref : Inport  Port=4
  Display2 : Display
  Memory1 : Memory  InheritSampleTime=on
  PI-reg. id : Subsystem
  PI-reg. iq : Subsystem
  PI-reg. w : Subsystem
  Saturation5 : Saturate  UpperLimit=Imax  LowerLimit=-Imax  OutDataType=fixdt(1, 16)  OutScaling=2^0
  Switch : Switch  Threshold=Umax * 0.95  OutDataType=fixdt(1, 16)  OutScaling=2^0  ZeroCross=off
  evaluation id_ref : Subsystem
  evaluation id_ref field-weakening : Subsystem
  id1 : InportShadow  Port=1  LatchByCopyingInsideSignal=off
  iq1 : InportShadow  Port=2  LatchByCopyingInsideSignal=off
  napetove omezeni menice : Subsystem
  "ud, uq to us" : Subsystem
  ud_lin to ud : Subsystem
  uq_lin to uq : Subsystem
  wm1 : InportShadow  Port=3  LatchByCopyingInsideSignal=off
  wm2 : InportShadow  Port=3  LatchByCopyingInsideSignal=off
  ud : Outport  OutDataType=fixdt(1, 16)  OutScaling=2^0
  uq : Outport  Port=2  OutDataType=fixdt(1, 16)  OutScaling=2^0
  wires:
  PI-reg. w/1(iq_ref) -> PI-reg. iq/1(iq_ref), evaluation id_ref/1(iq_ref)
  w_ref/1 -> PI-reg. w/1(w_ref)
  wm/1 -> PI-reg. w/2(wm)
  evaluation id_ref/1(id_ref) -> evaluation id_ref field-weakening/2(id_mtpa), Switch/3  "mtpa"
  "ud, uq to us"/1(us) -> Display2/1, Memory1/1
  [us] -> evaluation id_ref field-weakening/1(us), Switch/2
  id/1 -> PI-reg. id/2(id)
  iq1/1 -> ud_lin to ud/3(iq)
  iq/1 -> PI-reg. iq/2(iq)
  wm1/1 -> ud_lin to ud/2(wm)
  id1/1 -> uq_lin to uq/3(id)
  wm2/1 -> uq_lin to uq/2(wm)
  napetove omezeni menice/1(ud) -> ud/1
  napetove omezeni menice/2(uq) -> uq/1
  Memory1/1 -> [us]
  PI-reg. iq/1(uq1) -> uq_lin to uq/1(uq1)
  PI-reg. id/1(ud1) -> ud_lin to ud/1(ud1)
  ud_lin to ud/1(ud2) -> napetove omezeni menice/1(ud2), "ud, uq to us"/1(ud2)
  uq_lin to uq/1(uq2) -> napetove omezeni menice/2(uq2), "ud, uq to us"/2(uq2)
  evaluation id_ref field-weakening/1(id_ref) -> Switch/1
  Switch/1 -> Saturation5/1
  Saturation5/1 -> PI-reg. id/1(id_ref), PI-reg. w/3(id_ref)

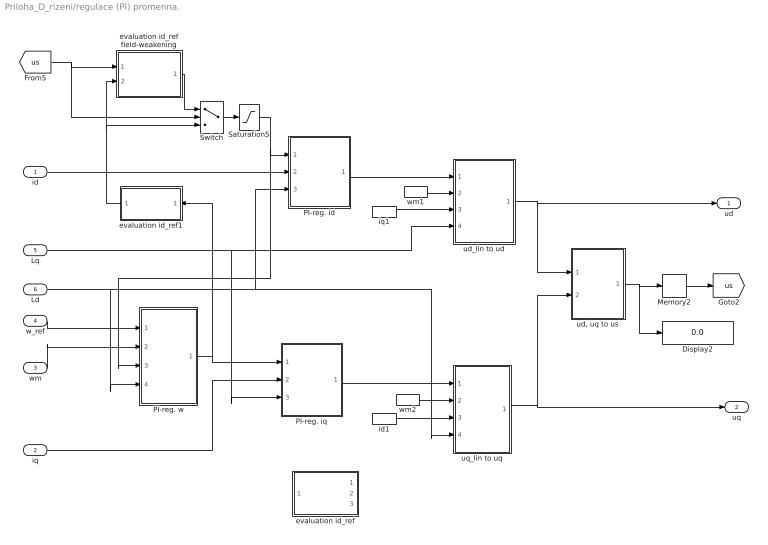
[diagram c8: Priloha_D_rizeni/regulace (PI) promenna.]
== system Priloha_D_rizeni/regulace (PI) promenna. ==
  id : Inport
  iq : Inport  Port=2
  wm : Inport  Port=3
  w_ref : Inport  Port=4
  Lq : Inport  Port=5
  Ld : Inport  Port=6
  Display2 : Display
  Memory2 : Memory  InheritSampleTime=on
  PI-reg. id : Subsystem
  PI-reg. iq : Subsystem
  PI-reg. w : Subsystem
  Saturation5 : Saturate  UpperLimit=Imax  LowerLimit=-Imax  OutDataType=fixdt(1, 16)  OutScaling=2^0
  Switch : Switch  Threshold=Umax * 0.95  OutDataType=fixdt(1, 16)  OutScaling=2^0  ZeroCross=off
  evaluation id_ref : Subsystem
  evaluation id_ref1 : Subsystem
  evaluation id_ref field-weakening : Subsystem
  id1 : InportShadow  Port=1  LatchByCopyingInsideSignal=off
  iq1 : InportShadow  Port=2  LatchByCopyingInsideSignal=off
  "ud, uq to us" : Subsystem
  ud_lin to ud : Subsystem
  uq_lin to uq : Subsystem
  wm1 : InportShadow  Port=3  LatchByCopyingInsideSignal=off
  wm2 : InportShadow  Port=3  LatchByCopyingInsideSignal=off
  ud : Outport  OutDataType=fixdt(1, 16)  OutScaling=2^0
  uq : Outport  Port=2  OutDataType=fixdt(1, 16)  OutScaling=2^0
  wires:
  PI-reg. w/1(iq_ref) -> evaluation id_ref1/1(iq_ref), PI-reg. iq/1(iq_ref)
  w_ref/1 -> PI-reg. w/1(w_ref)
  wm/1 -> PI-reg. w/2(wm)
  "ud, uq to us"/1(us) -> Display2/1, Memory2/1
  [us] -> evaluation id_ref field-weakening/1(us), Switch/2
  id/1 -> PI-reg. id/2(id)
  iq1/1 -> ud_lin to ud/3(iq)
  iq/1 -> PI-reg. iq/2(iq)
  wm1/1 -> ud_lin to ud/2(wm)
  id1/1 -> uq_lin to uq/3(id)
  wm2/1 -> uq_lin to uq/2(wm)
  PI-reg. id/1(ud_lin) -> ud_lin to ud/1(ud_lin)
  PI-reg. iq/1(uq_lin) -> uq_lin to uq/1(uq_lin)
  ud_lin to ud/1(ud1) -> ud/1, "ud, uq to us"/1(ud)
  uq_lin to uq/1(uq1) -> uq/1, "ud, uq to us"/2(uq)
  Lq/1 -> ud_lin to ud/4(Lq), PI-reg. iq/3(Lq)
  Ld/1 -> PI-reg. w/4(Ld), uq_lin to uq/4(Ld), PI-reg. id/3(Ld)
  evaluation id_ref field-weakening/1(id_ref) -> Switch/1
  Switch/1 -> Saturation5/1
  evaluation id_ref1/1(id_ref) -> Switch/3, evaluation id_ref field-weakening/2(id_mtpa)
  Memory2/1 -> [us]
  Saturation5/1 -> PI-reg. id/1(id_ref), PI-reg. w/3(id_ref)

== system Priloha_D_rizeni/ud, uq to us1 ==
  ud : Inport
  uq : Inport  Port=2
  Add3 : Sum  OutDataType=fixdt(1, 16)  OutScaling=2^-10
  Math Function : Math  Operator=magnitude^2  OutputSignalType=real  OutDataType=fixdt(1, 16)  OutScaling=2^0
  Math Function1 : Math  Operator=magnitude^2  OutputSignalType=real  OutDataType=fixdt(1, 16)  OutScaling=2^0
  Math Funtion2 : Math  Operator=sqrt  OutputSignalType=real  OutDataType=fixdt(1, 16)  OutScaling=2^0
  us : Outport
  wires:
  Math Function/1 -> Add3/1
  Math Function1/1 -> Add3/2
  Add3/1 -> Math Funtion2/1
  ud/1 -> Math Function/1
  Math Funtion2/1 -> us/1
  uq/1 -> Math Function1/1

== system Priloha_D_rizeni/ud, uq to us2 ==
  id : Inport
  iq : Inport  Port=2
  Add3 : Sum  OutDataType=fixdt(1, 16)  OutScaling=2^-10
  Math Function : Math  Operator=magnitude^2  OutputSignalType=real  OutDataType=fixdt(1, 16)  OutScaling=2^0
  Math Function1 : Math  Operator=magnitude^2  OutputSignalType=real  OutDataType=fixdt(1, 16)  OutScaling=2^0
  Math Funtion2 : Math  Operator=sqrt  OutputSignalType=real  OutDataType=fixdt(1, 16)  OutScaling=2^0
  is : Outport
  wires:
  iq/1 -> Math Function1/1
  Math Funtion2/1 -> is/1
  id/1 -> Math Function/1
  Add3/1 -> Math Funtion2/1
  Math Function1/1 -> Add3/2
  Math Function/1 -> Add3/1

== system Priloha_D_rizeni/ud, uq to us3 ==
  ud : Inport
  uq : Inport  Port=2
  Add3 : Sum  OutDataType=fixdt(1, 16)  OutScaling=2^-10
  Math Function : Math  Operator=magnitude^2  OutputSignalType=real  OutDataType=fixdt(1, 16)  OutScaling=2^0
  Math Function1 : Math  Operator=magnitude^2  OutputSignalType=real  OutDataType=fixdt(1, 16)  OutScaling=2^0
  Math Funtion2 : Math  Operator=sqrt  OutputSignalType=real  OutDataType=fixdt(1, 16)  OutScaling=2^0
  us : Outport
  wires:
  Math Function/1 -> Add3/1
  Math Function1/1 -> Add3/2
  Add3/1 -> Math Funtion2/1
  ud/1 -> Math Function/1
  Math Funtion2/1 -> us/1
  uq/1 -> Math Function1/1

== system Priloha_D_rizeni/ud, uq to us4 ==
  id : Inport
  iq : Inport  Port=2
  Add3 : Sum  OutDataType=fixdt(1, 16)  OutScaling=2^-10
  Math Function : Math  Operator=magnitude^2  OutputSignalType=real  OutDataType=fixdt(1, 16)  OutScaling=2^0
  Math Function1 : Math  Operator=magnitude^2  OutputSignalType=real  OutDataType=fixdt(1, 16)  OutScaling=2^0
  Math Funtion2 : Math  Operator=sqrt  OutputSignalType=real  OutDataType=fixdt(1, 16)  OutScaling=2^0
  is : Outport
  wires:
  iq/1 -> Math Function1/1
  Math Funtion2/1 -> is/1
  id/1 -> Math Function/1
  Add3/1 -> Math Funtion2/1
  Math Function1/1 -> Add3/2
  Math Function/1 -> Add3/1

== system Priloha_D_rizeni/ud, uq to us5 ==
  ud : Inport
  uq : Inport  Port=2
  Add3 : Sum  OutDataType=fixdt(1, 16)  OutScaling=2^-10
  Math Function : Math  Operator=magnitude^2  OutputSignalType=real  OutDataType=fixdt(1, 16)  OutScaling=2^0
  Math Function1 : Math  Operator=magnitude^2  OutputSignalType=real  OutDataType=fixdt(1, 16)  OutScaling=2^0
  Math Funtion2 : Math  Operator=sqrt  OutputSignalType=real  OutDataType=fixdt(1, 16)  OutScaling=2^0
  us : Outport
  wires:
  Math Function/1 -> Add3/1
  Math Function1/1 -> Add3/2
  Add3/1 -> Math Funtion2/1
  ud/1 -> Math Function/1
  Math Funtion2/1 -> us/1
  uq/1 -> Math Function1/1

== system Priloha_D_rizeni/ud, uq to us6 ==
  id : Inport
  iq : Inport  Port=2
  Add3 : Sum  OutDataType=fixdt(1, 16)  OutScaling=2^-10
  Math Function : Math  Operator=magnitude^2  OutputSignalType=real  OutDataType=fixdt(1, 16)  OutScaling=2^0
  Math Function1 : Math  Operator=magnitude^2  OutputSignalType=real  OutDataType=fixdt(1, 16)  OutScaling=2^0
  Math Funtion2 : Math  Operator=sqrt  OutputSignalType=real  OutDataType=fixdt(1, 16)  OutScaling=2^0
  is : Outport
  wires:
  iq/1 -> Math Function1/1
  Math Funtion2/1 -> is/1
  id/1 -> Math Function/1
  Add3/1 -> Math Funtion2/1
  Math Function1/1 -> Add3/2
  Math Function/1 -> Add3/1

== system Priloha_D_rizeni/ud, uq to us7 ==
  ud : Inport
  uq : Inport  Port=2
  Add3 : Sum  OutDataType=fixdt(1, 16)  OutScaling=2^-10
  Math Function : Math  Operator=magnitude^2  OutputSignalType=real  OutDataType=fixdt(1, 16)  OutScaling=2^0
  Math Function1 : Math  Operator=magnitude^2  OutputSignalType=real  OutDataType=fixdt(1, 16)  OutScaling=2^0
  Math Funtion2 : Math  Operator=sqrt  OutputSignalType=real  OutDataType=fixdt(1, 16)  OutScaling=2^0
  us : Outport
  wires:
  Math Function/1 -> Add3/1
  Math Function1/1 -> Add3/2
  Add3/1 -> Math Funtion2/1
  ud/1 -> Math Function/1
  Math Funtion2/1 -> us/1
  uq/1 -> Math Function1/1

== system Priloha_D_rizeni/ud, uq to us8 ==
  id : Inport
  iq : Inport  Port=2
  Add3 : Sum  OutDataType=fixdt(1, 16)  OutScaling=2^-10
  Math Function : Math  Operator=magnitude^2  OutputSignalType=real  OutDataType=fixdt(1, 16)  OutScaling=2^0
  Math Function1 : Math  Operator=magnitude^2  OutputSignalType=real  OutDataType=fixdt(1, 16)  OutScaling=2^0
  Math Funtion2 : Math  Operator=sqrt  OutputSignalType=real  OutDataType=fixdt(1, 16)  OutScaling=2^0
  is : Outport
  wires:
  iq/1 -> Math Function1/1
  Math Funtion2/1 -> is/1
  id/1 -> Math Function/1
  Add3/1 -> Math Funtion2/1
  Math Function1/1 -> Add3/2
  Math Function/1 -> Add3/1

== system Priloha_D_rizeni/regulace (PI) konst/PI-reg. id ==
  note: PI-regulator proudu id
  id_ref : Inport
  id : Inport  Port=2
  Add : Sum  OutDataType=fixdt(1, 16)  OutScaling=2^-10
  Add1 : Sum  Inputs=+-  OutDataType=fixdt(1, 16)  OutScaling=2^-10
  I : Gain  Gain=Kiid  ParameterDataType=fixdt(1, 16)  ParameterScaling=2^0  OutDataType=fixdt(1, 16)  OutScaling=2^0
  Integrator1 : Integrator  LimitOutput=on  UpperSaturationLimit=Umax  LowerSaturationLimit=-Umax
  P2 : Gain  Gain=Kpid  ParameterDataType=fixdt(1, 16)  ParameterScaling=2^0  OutDataType=fixdt(1, 16)  OutScaling=2^0
  ud1 : Outport
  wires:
  P2/1 -> Add/1
  Integrator1/1 -> Add/2
  Add/1 -> ud1/1
  id_ref/1 -> Add1/1
  id/1 -> Add1/2
  I/1 -> Integrator1/1
  Add1/1 -> I/1, P2/1

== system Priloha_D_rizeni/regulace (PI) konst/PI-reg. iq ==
  note: PI-regulator proudu iq
  iq_ref : Inport
  iq : Inport  Port=2
  Add : Sum  OutDataType=fixdt(1, 16)  OutScaling=2^-10
  Add1 : Sum  Inputs=+-  OutDataType=fixdt(1, 16)  OutScaling=2^-10
  I : Gain  Gain=Kiiq  ParameterDataType=fixdt(1, 16)  ParameterScaling=2^0  OutDataType=fixdt(1, 16)  OutScaling=2^0
  Integrator1 : Integrator  LimitOutput=on  UpperSaturationLimit=Umax  LowerSaturationLimit=-Umax
  P : Gain  Gain=Kpiq  ParameterDataType=fixdt(1, 16)  ParameterScaling=2^0  OutDataType=fixdt(1, 16)  OutScaling=2^0
  uq1 : Outport
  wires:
  Integrator1/1 -> Add/2
  P/1 -> Add/1
  iq_ref/1 -> Add1/1
  iq/1 -> Add1/2
  Add/1 -> uq1/1
  I/1 -> Integrator1/1
  Add1/1 -> P/1, I/1

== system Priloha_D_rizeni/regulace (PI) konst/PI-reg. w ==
  note: PI-regulator otacek
  w_ref : Inport
  wm : Inport  Port=2
  id_ref : Inport  Port=3
  Add : Sum  OutDataType=fixdt(1, 16)  OutScaling=2^-10
  Add2 : Sum  Inputs=+-  OutDataType=fixdt(1, 16)  OutScaling=2^-10
  Add3 : Sum  Inputs=+-  OutDataType=fixdt(1, 16)  OutScaling=2^-10
  I : Gain  Gain=Kiwq  ParameterDataType=fixdt(1, 16)  ParameterScaling=2^0  OutDataType=fixdt(1, 16)  OutScaling=2^0
  I1 : Gain  Gain=-1  ParameterDataType=fixdt(1, 16)  ParameterScaling=2^0  OutDataType=fixdt(1, 16)  OutScaling=2^0
  Integrator1 : Integrator  LimitOutput=on  UpperSaturationLimit=Imax  LowerSaturationLimit=-Imax
  Math Function : Math  Operator=magnitude^2  OutputSignalType=real  OutDataType=fixdt(1, 16)  OutScaling=2^0
  Math Funtion2 : Math  Operator=sqrt  OutputSignalType=real  OutDataType=fixdt(1, 16)  OutScaling=2^0
  P : Gain  Gain=Kpwq  ParameterDataType=fixdt(1, 16)  ParameterScaling=2^0  OutDataType=fixdt(1, 16)  OutScaling=2^0
  Saturation Dynamic : Subsystem  AncestorBlock=simulink/Discontinuities/Saturation Dynamic  mask(Saturation Dynamic){OutMin=[], OutMax=[], OutDataTypeStr=Inherit: Same as second input, OutputDataTypeScalingMode=Same as second input, OutDataType=fixdt(1, 16), OutScaling=2^-10, LockScale=off, RndMeth=Floor, DoSatur=off}
      mask prompts: OutMin "Output minimum:"; OutMax "Output maximum:"; OutDataTypeStr "Output data type:"; OutputDataTypeScalingMode "Output data type mode:"; OutDataType "Output data type (e.g. fixdt(1, 16), fixdt('single')):"; OutScaling "Output scaling (Slope, e.g. 2^-9 or [Slope Bias], e.g. [1.25 3]):"; LockScale "Lock output scaling against changes by the autoscaling tool"; RndMeth "Integer rounding mode:"; DoSatur "Saturate on integer overflow"
      mask help: Bound the range of the second input by using the first input (upper limit) and the third input (lower limit).
      mask init:
      | blkH = gcbh;
      | blkName = getfullname(blkH);
      | 
      | switch_blks = {'Switch','Switch2'}; 
      | for i = 1:length(switch_blks)
      |   set_param([blkName,'/',switch_blks{i}], ...
      |       'RndMeth', RndMeth, ...
      | 	  'DoSatur', DoSatur);
      | end
      | 
      | propBlk = [blkName, '/Data Type Propagation'];
      | 
      | if strcmp(OutputDataTypeScalingMode, 'Same as second input')
      |     set_param(propBlk, 'PropDataTypeMode', 'Inherit via propagation rule', ...
      |                        'PropScalingMode',  'Inherit via propagation rule');
      | else
      |     scaling = OutScaling;
      |     switch OutputDataTypeScalingMode
      |       case 'double'
      |         dataType = 'fixdt(''double'')';
      |       case 'single'
      |         dataType = 'fixdt(''single'')';
      |       case 'int8'
      |         dataType = 'fixdt(1,8,0)';
      |       case 'uint8'
      |         dataType = 'fixdt(0,8,0)';
      |       case 'int16'
      |         dataType = 'fixdt(1,16,0)';
      |       case 'uint16'
      |         dataType = 'fixdt(0,16,0)';
      |       case 'int32'
      |         dataType = 'fixdt(1,32,0)';
      |       case 'uint32'
      |         dataType = 'fixdt(0,32,0)';
      |       case 'Specify via dialog'
      |         dataType = OutDataType;
      |     end
      |     
      |     set_param(propBlk, 'PropDataTypeMode', 'Specify via dialog', ...
      |                        'PropScalingMode',  'Specify via dialog', ...
      |                        'PropDataType',     dataType, ...
      |                        'PropScaling',      scaling);
      | end
  id_ref4 : Constant  Value=Imax^2  OutDataType=fixdt(1, 16)  OutScaling=2^0
  iq_ref : Outport
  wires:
  P/1 -> Add/1
  Integrator1/1 -> Add/2
  Add/1 -> Saturation Dynamic/2(u)
  w_ref/1 -> Add2/1
  wm/1 -> Add2/2
  Add2/1 -> P/1, I/1
  Saturation Dynamic/1(y1) -> iq_ref/1
  I/1 -> Integrator1/1
  id_ref/1 -> Math Function/1
  Add3/1 -> Math Funtion2/1
  Math Funtion2/1 -> Saturation Dynamic/1(up), I1/1
  Math Function/1 -> Add3/2
  id_ref4/1 -> Add3/1
  I1/1 -> Saturation Dynamic/3(lo)

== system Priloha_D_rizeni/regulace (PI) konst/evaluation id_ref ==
  iq_ref : Inport
  Add3 : Sum  OutDataType=fixdt(1, 16)  OutScaling=2^-10
  Add4 : Sum  Inputs=+-  OutDataType=fixdt(1, 16)  OutScaling=2^-10
  Divide : Product  Inputs=*/  OutDataType=fixdt(1, 16)  OutScaling=2^-10
  Divide1 : Product  Inputs=*/  OutDataType=fixdt(1, 16)  OutScaling=2^-10
  Gain : Gain  Gain=4  ParameterDataType=fixdt(1, 16)  ParameterScaling=2^0  OutDataType=fixdt(1, 16)  OutScaling=2^0
  Gain1 : Gain  Gain=2  ParameterDataType=fixdt(1, 16)  ParameterScaling=2^0  OutDataType=fixdt(1, 16)  OutScaling=2^0
  Math Function : Math  Operator=magnitude^2  OutputSignalType=real  OutDataType=fixdt(1, 16)  OutScaling=2^0
  Math Function1 : Math  Operator=magnitude^2  OutputSignalType=real  OutDataType=fixdt(1, 16)  OutScaling=2^0
  Math Function2 : Math  Operator=magnitude^2  OutputSignalType=real  OutDataType=fixdt(1, 16)  OutScaling=2^0
  Math Function3 : Math  Operator=sqrt  OutputSignalType=real  OutDataType=fixdt(1, 16)  OutScaling=2^0
  w_ref1 : Constant  Value=Lq - Ld  OutDataType=fixdt(1, 16)  OutScaling=2^0
  w_ref2 : Constant  Value=Psim  OutDataType=fixdt(1, 16)  OutScaling=2^0
  id_ref : Outport
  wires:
  Math Function/1 -> Add3/2
  w_ref2/1 -> Math Function1/1, Divide1/1
  Math Function1/1 -> Divide/1
  Math Function2/1 -> Gain/1
  Divide/1 -> Add3/1
  Add3/1 -> Math Function3/1
  Divide1/1 -> Add4/1
  w_ref1/1 -> Math Function2/1, Gain1/1
  Math Function3/1 -> Add4/2
  Gain/1 -> Divide/2
  Gain1/1 -> Divide1/2
  iq_ref/1 -> Math Function/1
  Add4/1 -> id_ref/1
